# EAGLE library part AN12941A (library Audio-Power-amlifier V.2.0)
Audio power IC for notebook PC
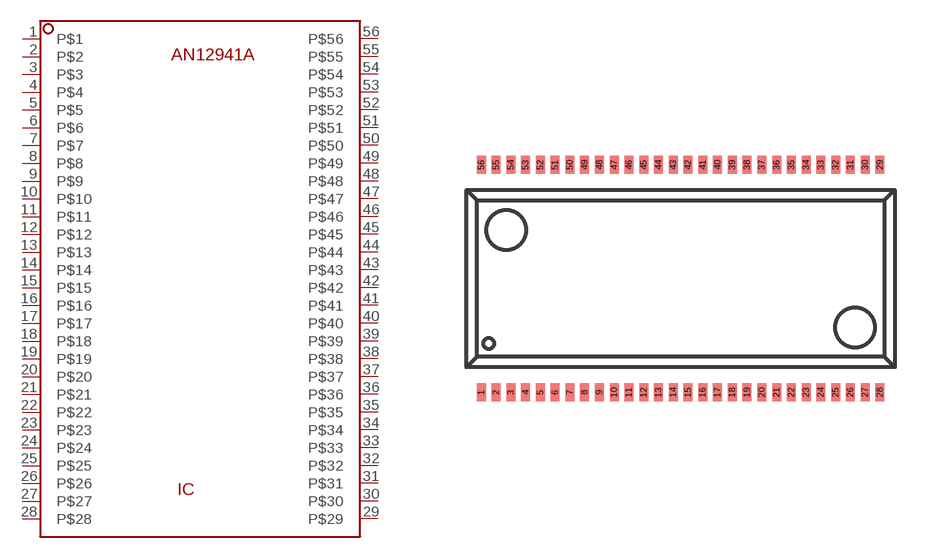
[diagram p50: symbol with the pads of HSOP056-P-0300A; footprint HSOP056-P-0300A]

Designator prefix IC

## AN12941A  [HSOP056-P-0300A]
1  P$1  pwr
2  P$2
3  P$3
4  P$4  in
5  P$5
6  P$6
7  P$7
8  P$8
9  P$9
10  P$10
11  P$11
12  P$12
13  P$13
14  P$14
15  P$15  pwr
16  P$16  in
17  P$17
18  P$18
19  P$19
20  P$20  pwr
21  P$21
22  P$22
23  P$23  pwr
24  P$24  out
25  P$25  out
26  P$26  out
27  P$27  out
28  P$28  pwr
29  P$29  pwr
30  P$30  out
31  P$31  out
32  P$32  out
33  P$33  out
34  P$34  pwr
35  P$35
36  P$36
37  P$37  pwr
38  P$38
39  P$39  out
40  P$40
41  P$41  in
42  P$42  pwr
43  P$43  out
44  P$44  out
45  P$45
46  P$46  out
47  P$47  in
48  P$48  out
49  P$49  out
50  P$50  in
51  P$51  out
52  P$52  in
53  P$53
54  P$54  in
55  P$55  pwr
56  P$56  in

## Footprint HSOP056-P-0300A (pad centres in mm)
smd 0.305 x 0.61: 1 -7,-3.85; 2 -6.5,-3.85; 3 -6,-3.85; 4 -5.5,-3.85; 5 -5,-3.85; 6 -4.5,-3.85; 7 -4,-3.85; 8 -3.5,-3.85; 9 -3,-3.85; 10 -2.5,-3.85; 11 -2,-3.85; 12 -1.5,-3.85; 13 -1,-3.85; 14 -0.5,-3.85; 15 0,-3.85; 16 0.5,-3.85; 17 1,-3.85; 18 1.5,-3.85; 19 2,-3.85; 20 2.5,-3.85; 21 3,-3.85; 22 3.5,-3.85; 23 4,-3.85; 24 4.5,-3.85; 25 5,-3.85; 26 5.5,-3.85; 27 6,-3.85; 28 6.5,-3.85; 29 6.5,3.85; 30 6,3.85; 31 5.5,3.85; 32 5,3.85; 33 4.5,3.85; 34 4,3.85; 35 3.5,3.85; 36 3,3.85; 37 2.5,3.85; 38 2,3.85; 39 1.5,3.85; 40 1,3.85; 41 0.5,3.85; 42 0,3.85; 43 -0.5,3.85; 44 -1,3.85; 45 -1.5,3.85; 46 -2,3.85; 47 -2.5,3.85; 48 -3,3.85; 49 -3.5,3.85; 50 -4,3.85; 51 -4.5,3.85; 52 -5,3.85; 53 -5.5,3.85; 54 -6,3.85; 55 -6.5,3.85; 56 -7,3.85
